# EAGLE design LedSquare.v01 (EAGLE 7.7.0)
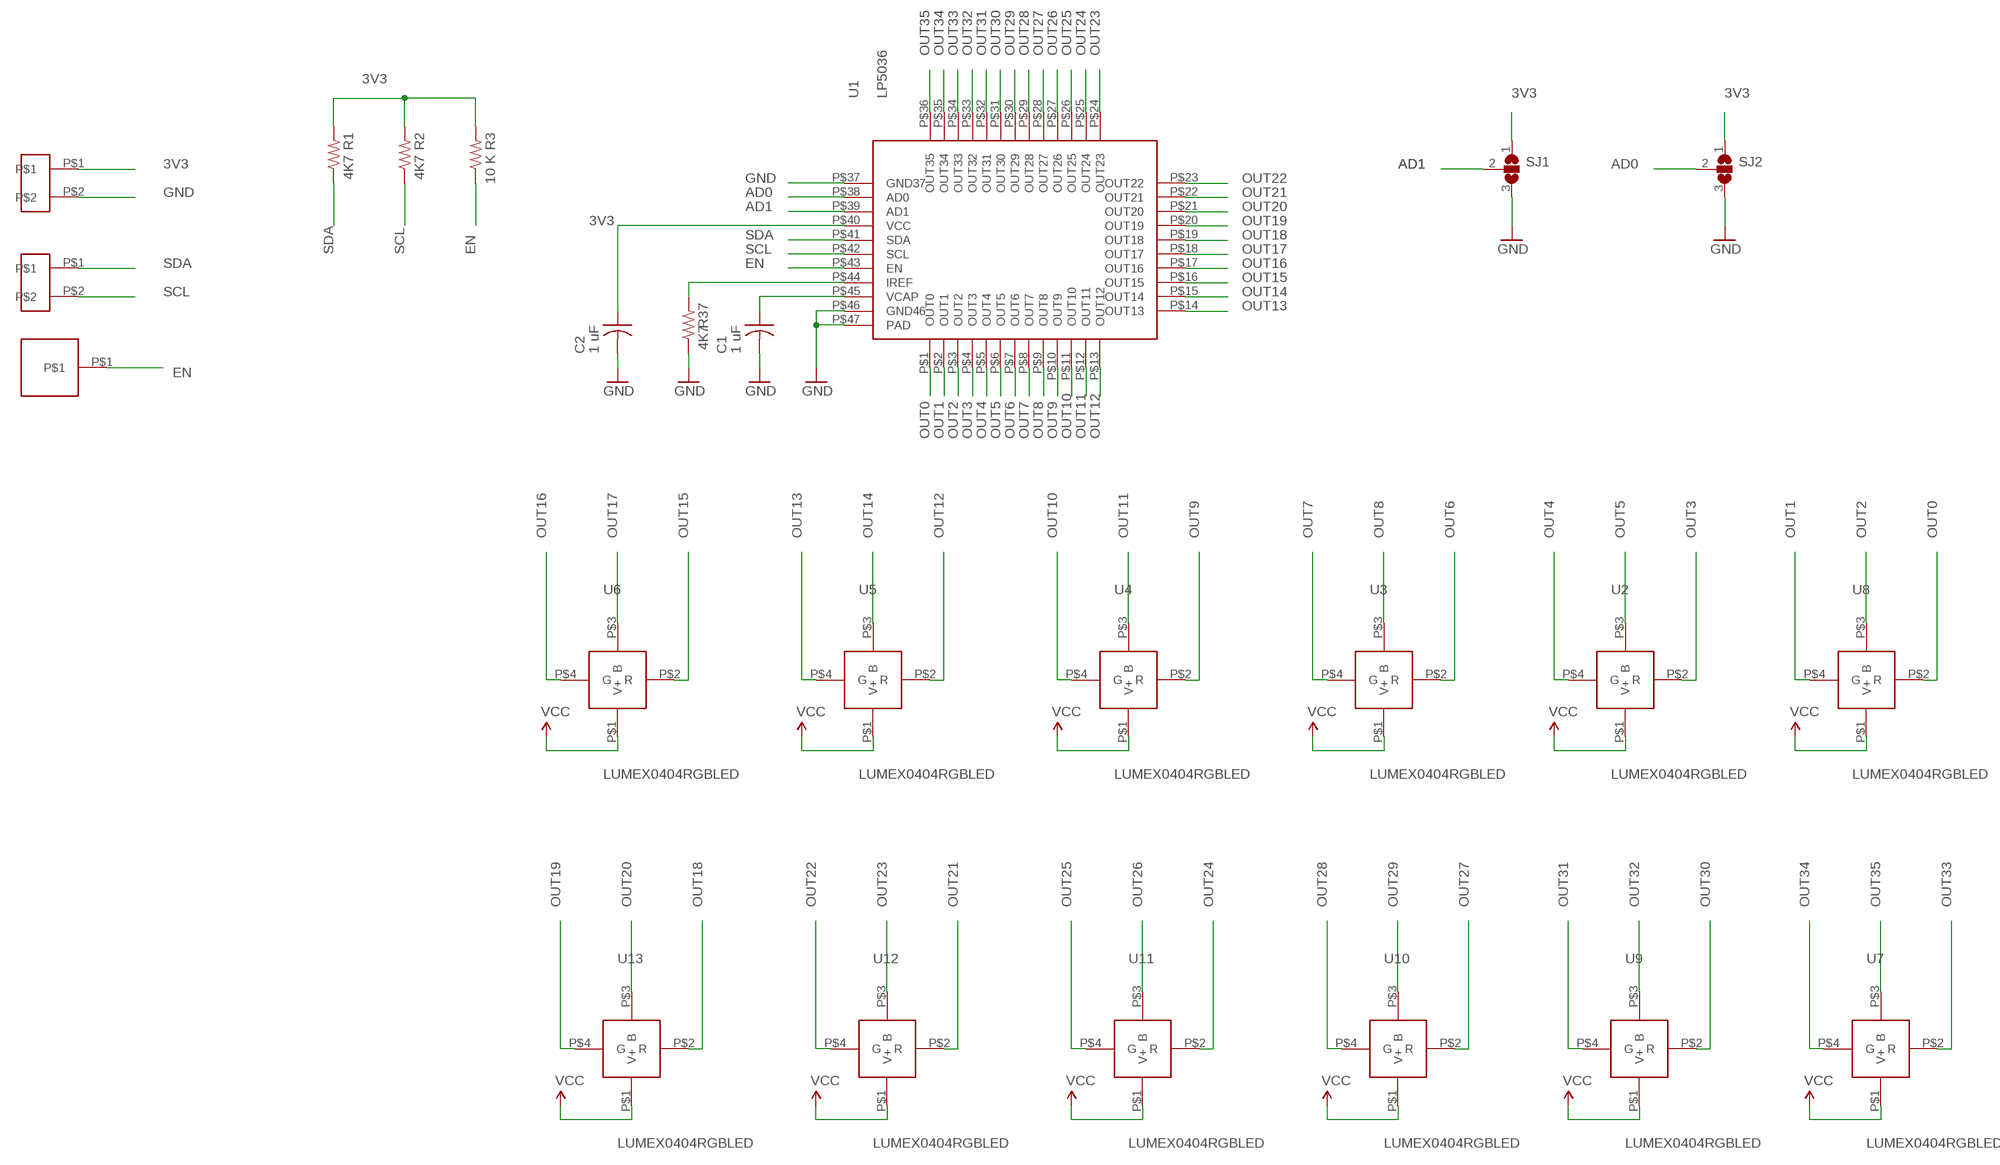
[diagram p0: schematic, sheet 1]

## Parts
C1  1 uF  C-US  [C0402_B]
C2  1 uF  C-US  [C0402_B]
R1  4K7  R-US_  [R0402_B]
R2  4K7  R-US_  [R0402_B]
R3  10 K  R-US_  [R0402_B]
R37  4K7  R-US_  [R0402_B]
SJ1  SJ2W  [SJ_2]
SJ2  SJ2W  [SJ_2]
U1  LP5036  [LP5036]
U2  LUMEX0404RGBLED  [LX0404]
U3  LUMEX0404RGBLED  [LX0404]
U4  LUMEX0404RGBLED  [LX0404]
U5  LUMEX0404RGBLED  [LX0404]
U6  LUMEX0404RGBLED  [LX0404]
U7  LUMEX0404RGBLED  [LX0404]
U8  LUMEX0404RGBLED  [LX0404]
U9  LUMEX0404RGBLED  [LX0404]
U10  LUMEX0404RGBLED  [LX0404]
U11  LUMEX0404RGBLED  [LX0404]
U12  LUMEX0404RGBLED  [LX0404]
U13  LUMEX0404RGBLED  [LX0404]
U$9  HN01  [HN01]
U$17  HN02  [HN02]
U$39  HN02  [HN02]

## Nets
3V3: C2.1 R1.2 R2.2 R3.2 SJ1.1 SJ2.1 U1.P$40(VCC) U2.P$1(V+) U3.P$1(V+) U4.P$1(V+) U5.P$1(V+) U6.P$1(V+) U7.P$1(V+) U8.P$1(V+) U9.P$1(V+) U10.P$1(V+) U11.P$1(V+) U12.P$1(V+) U13.P$1(V+) U$39.P$1 ; supply symbol labelled VCC
AD0: SJ2.2 U1.P$38(AD0)
AD1: SJ1.2 U1.P$39(AD1)
EN: R3.1 U1.P$43(EN) U$9.P$1
GND: C1.2 C2.2 R37.1 SJ1.3 SJ2.3 U1.P$37(GND37) U1.P$46(GND46) U1.P$47(PAD) U$39.P$2
N$80: R37.2 U1.P$44(IREF)
N$81: C1.1 U1.P$45(VCAP)
OUT0: U1.P$1(OUT0) U8.P$2(R)
OUT1: U1.P$2(OUT1) U8.P$4(G)
OUT2: U1.P$3(OUT2) U8.P$3(B)
OUT3: U1.P$4(OUT3) U2.P$2(R)
OUT4: U1.P$5(OUT4) U2.P$4(G)
OUT5: U1.P$6(OUT5) U2.P$3(B)
OUT6: U1.P$7(OUT6) U3.P$2(R)
OUT7: U1.P$8(OUT7) U3.P$4(G)
OUT8: U1.P$9(OUT8) U3.P$3(B)
OUT9: U1.P$10(OUT9) U4.P$2(R)
OUT10: U1.P$11(OUT10) U4.P$4(G)
OUT11: U1.P$12(OUT11) U4.P$3(B)
OUT12: U1.P$13(OUT12) U5.P$2(R)
OUT13: U1.P$14(OUT13) U5.P$4(G)
OUT14: U1.P$15(OUT14) U5.P$3(B)
OUT15: U1.P$16(OUT15) U6.P$2(R)
OUT16: U1.P$17(OUT16) U6.P$4(G)
OUT17: U1.P$18(OUT17) U6.P$3(B)
OUT18: U1.P$19(OUT18) U13.P$2(R)
OUT19: U1.P$20(OUT19) U13.P$4(G)
OUT20: U1.P$21(OUT20) U13.P$3(B)
OUT21: U1.P$22(OUT21) U12.P$2(R)
OUT22: U1.P$23(OUT22) U12.P$4(G)
OUT23: U1.P$24(OUT23) U12.P$3(B)
OUT24: U1.P$25(OUT24) U11.P$2(R)
OUT25: U1.P$26(OUT25) U11.P$4(G)
OUT26: U1.P$27(OUT26) U11.P$3(B)
OUT27: U1.P$28(OUT27) U10.P$2(R)
OUT28: U1.P$29(OUT28) U10.P$4(G)
OUT29: U1.P$30(OUT29) U10.P$3(B)
OUT30: U1.P$31(OUT30) U9.P$2(R)
OUT31: U1.P$32(OUT31) U9.P$4(G)
OUT32: U1.P$33(OUT32) U9.P$3(B)
OUT33: U1.P$34(OUT33) U7.P$2(R)
OUT34: U1.P$35(OUT34) U7.P$4(G)
OUT35: U1.P$36(OUT35) U7.P$3(B)
SCL: R2.1 U1.P$42(SCL) U$17.P$2
SDA: R1.1 U1.P$41(SDA) U$17.P$1

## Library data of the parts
C1 C2 = Spark:C-US: Capacitor
R1-R3 R37 = Spark:R-US_: 0402 Resistor
SJ1 SJ2 = jumper:SJ2W: SMD solder JUMPER
U1 = Kris:LP5036: LP5036RJVR 12 x 3 rgb led driver http://www.ti.com/lit/ds/symlink/lp5036.pdf
U2-U13 = Kris:LUMEX0404RGBLED: Lumex 0404 rgb leds
U$9 = PWSONN6:HN01
U$17 U$39 = Kris:HN02: 0.1 inch header

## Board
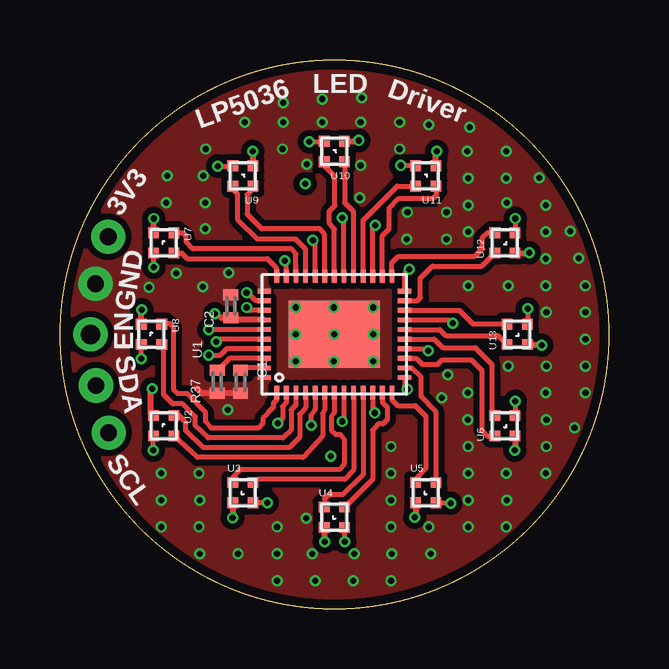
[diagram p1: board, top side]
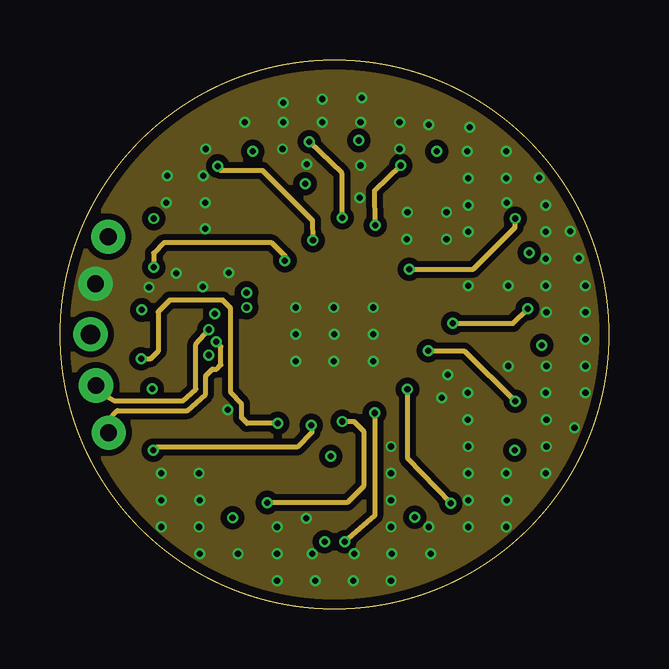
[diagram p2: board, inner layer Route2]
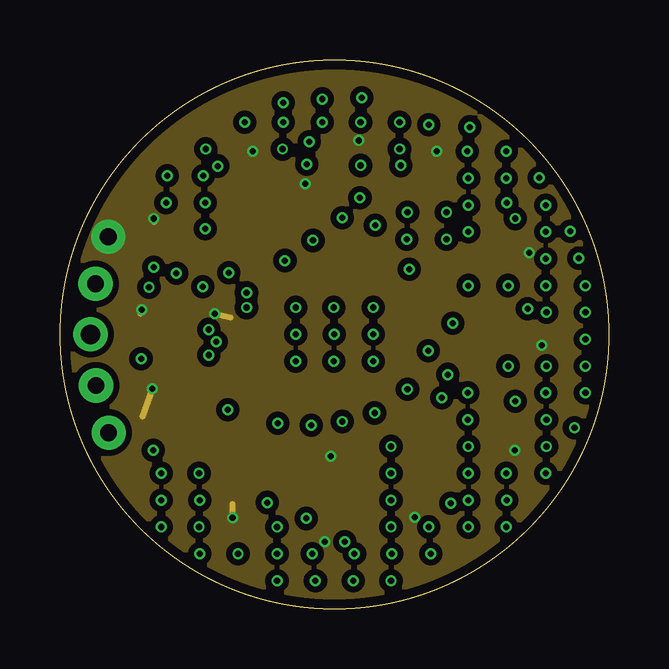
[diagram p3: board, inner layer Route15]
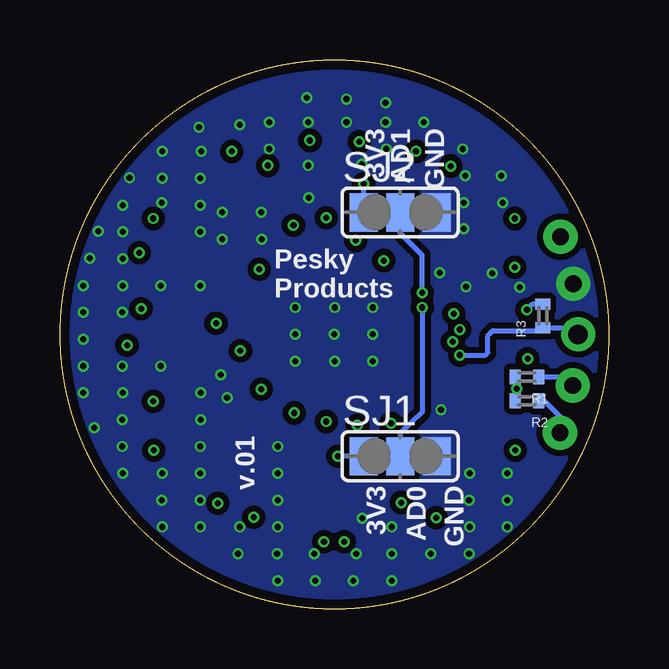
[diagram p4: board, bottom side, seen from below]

Size 22.86 x 22.86 mm. Coordinates in mm from the lower left corner, seen from the top.
Outline: circle at 11.43,11.43 radius 11.43
Copper layers (1*2*15*16): Top 0.035559375mm / dielectric 0.17018125mm / Route2 0.01778125mm / dielectric 47mil / Route15 0.01778125mm / dielectric 0.17018125mm / Bottom 0.035559375mm
Design rules "OSHPark-4layer *": minimum track width 5mil, minimum drill 10mil, track to track 5mil, track to pad 5mil, pad to pad 5mil, via to via 5mil, smd to smd 5mil, copper to edge 15mil, drill to drill 6mil, minimum pad ring 4mil, minimum via ring 4mil, stop-mask expansion 4mil, vias tented up to drill 20mil, thermal gap 10mil

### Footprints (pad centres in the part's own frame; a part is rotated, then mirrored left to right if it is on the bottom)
C0402_B = smd 0.457 x 0.61: 1 -0.483,0; 2 0.483,0
R0402_B = smd 0.457 x 0.61: 1 -0.483,0; 2 0.483,0
SJ_2 = smd 1.168 x 1.6: 1 -1.524,0; 2 0,0; 3 1.524,0
LP5036 = smd 0.55 x 0.2: P$1 -2.425,2.4; P$2 -2.425,2; P$3 -2.425,1.6; P$4 -2.425,1.2; P$5 -2.425,0.8; P$6 -2.425,0.4; P$7 -2.425,0; P$8 -2.425,-0.4; P$9 -2.425,-0.8; P$10 -2.425,-1.2; P$11 -2.425,-1.6; P$12 -2.425,-2; P$13 -2.425,-2.4; P$24 2.425,-2.4; P$25 2.425,-2; P$26 2.425,-1.6; P$27 2.425,-1.2; P$28 2.425,-0.8; P$29 2.425,-0.4; P$30 2.425,0; P$31 2.425,0.4; P$32 2.425,0.8; P$33 2.425,1.2; P$34 2.425,1.6; P$35 2.425,2; P$36 2.425,2.4 | smd 0.2 x 0.55: P$14 -1.8,-2.925; P$15 -1.4,-2.925; P$16 -1,-2.925; P$17 -0.6,-2.925; P$18 -0.2,-2.925; P$19 0.2,-2.925; P$20 0.6,-2.925; P$21 1,-2.925; P$22 1.4,-2.925; P$23 1.8,-2.925; P$37 1.8,2.925; P$38 1.4,2.925; P$39 1,2.925; P$40 0.6,2.925; P$41 0.2,2.925; P$42 -0.2,2.925; P$43 -0.6,2.925; P$44 -1,2.925; P$45 -1.4,2.925; P$46 -1.8,2.925 | smd 2.8 x 3.8: P$47 0,0
LX0404 = smd 0.45 x 0.45: P$1 -0.425,-0.425; P$2 -0.425,0.425; P$3 0.425,0.425; P$4 0.425,-0.425
HN01 = drill 0.813 pad 1.422: P$1 0,0
HN02 = drill 0.7 pad 1.422: P$1 0,0; P$2 -2.032,0

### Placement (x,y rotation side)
C1  7.52,9.45 270 top
C2  7.11,12.6 90 top
R1  3.4,9.65 180 bottom
R2  3.4,8.66 180 bottom
R3  2.74,12.19 90 bottom
R37  6.55,9.45 90 top
SJ1  8.69,6.35 0 bottom
SJ2  8.69,16.51 0 bottom
U1  11.43,11.43 90 top
U2  4.32,7.62 270 top
U3  7.62,4.83 0 top
U4  11.43,3.81 0 top
U5  15.24,4.83 0 top
U6  18.54,7.62 90 top
U7  4.32,15.24 270 top
U8  3.81,11.43 270 top
U9  7.62,18.03 180 top
U10  11.43,19.05 180 top
U11  15.24,18.03 180 top
U12  18.54,15.24 90 top
U13  19.05,11.43 90 top
U$9  1.27,11.43 0 top
U$17  1.5,9.3 105 top
U$39  2.01,15.49 75 top

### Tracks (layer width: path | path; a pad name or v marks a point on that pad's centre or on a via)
3V3  (via drill 0.25)
  Top 0.254: U1.P$40 7.23,12.03 C2.1 6.73,12.12 v6.45,12.29 | U9.P$1 8.04,19.03 v8.03,19.05 | U10.P$1 12.53,19.48 v12.45,19.51 | U11.P$1 15.66,18.98 v15.7,19.05 | U12.P$1 19.49,14.82 v19.56,14.83 | U13.P$1 20.03,11.01 v20.07,10.97 | U6.P$1 18.96,6.62 v18.95,6.6 | U5.P$1 14.82,3.88 v14.78,3.81 | U4.P$1 11.01,2.86 v11.02,2.79 | U8.P$1 3.39,12.43 v3.4,12.45 | U7.P$1 3.9,16.14 v3.91,16.26 | U3.P$1 7.2,3.74 v7.19,3.79 | U2.P$1 3.87,8.04 3.79,8.13 3.79,9.11 v3.84,9.16
  Route15 0.203: v11.28,6.35 11.38,6.4
  Route15 0.254: v6.45,12.29 7.11,12.14 | v8.03,19.05 8.03,19.1 8.08,19.05 | v12.45,19.51 12.39,19.46 12.34,19.51 | v15.7,19.05 15.65,18.95 | v19.56,14.83 19.51,14.83 | v20.07,10.97 19.96,10.97 20.02,11.02 | v18.95,6.6 18.95,6.71 | v14.78,3.81 14.83,3.86 14.78,3.91 | v11.02,2.79 10.97,2.79 | v3.84,9.16 3.43,8 | v3.4,12.45 3.45,12.39 3.35,12.29 | v3.91,16.26 3.96,16.15 3.91,16.1 | v7.19,3.79 7.19,4.37
  Bottom 0.203: SJ2.1 v10.21,17.7 | SJ1.1 v11.28,6.35 11.38,6.35 | R3.2 3.18,12.68 v3.4,12.45 | R2.2 3.86,9.13 v3.84,9.16
  Bottom 0.254: R1.2 R2.2
  pour Route15 (isolate 0.254, no thermals): -1.27,24.13 24.13,24.13 24.13,-1.27 -1.27,-1.27
AD0  (via drill 0.25)
  Top 0.203: U1.P$38 8.15,12.83 7.82,13.16 v7.77,13.16
  Bottom 0.203: v7.77,13.16 7.77,14.73 8.69,15.65 SJ2.2
AD1  (via drill 0.25)
  Top 0.203: U1.P$39 7.94,12.43 v7.77,12.55
  Bottom 0.127: SJ1.2 7.21,6.35
  Bottom 0.203: v7.77,12.55 7.77,8.18 8.69,7.32 SJ1.2
EN  (via drill 0.25)
  Top 0.203: U1.P$43 6.94,10.83 6.68,10.57 v6.2,10.57
  Bottom 0.203: v6.2,10.57 5.13,10.57 5.03,10.67 5.03,11.38 4.83,11.58 2.95,11.58 R3.1 1.55,11.71 U$9.P$1
GND  (via drill 0.25)
  Top 0.254: C1.2 5.92,8.97 5.72,9.17
  other vias: 11.43,11.43 6.99,8.28 9.83,12.55 11.4,12.55 13.06,12.55 13.06,10.31 13.06,11.43 11.4,10.31 9.83,10.31 9.83,11.43 5.82,4.52 4.22,5.64 5.79,5.64 5.79,3.4 4.22,3.4 4.22,4.52 7.42,2.29 9.04,3.4 9.04,1.17 9.04,2.29 5.82,2.29 10.64,1.17 10.52,2.29 12.27,2.29 13.82,2.29 13.79,3.4 15.44,2.29 13.79,1.17 12.22,1.17 13.79,5.64 17.02,5.64 17.02,3.4 17.02,4.52 15.37,3.4 13.79,4.52 13.79,6.76 17.02,6.76 18.62,4.52 18.59,5.64 20.24,5.64 18.59,3.4 16.99,8.99 20.27,6.76 20.27,7.87 16.99,7.87 20.27,10.11 21.89,11.23 21.89,8.99 21.89,10.11 20.24,8.99 18.67,10.11 20.27,12.34 18.67,13.46 20.24,13.46 21.89,13.46 21.89,12.34 16.15,9.75 15.9,8.79 17.02,15.7 20.24,15.7 20.24,14.58 17.02,13.46 18.62,16.92 17.02,17.93 18.59,17.93 20.24,16.81 17.02,16.81 16.97,19.05 15.37,20.17 17.07,20.07 18.59,19.05 19.96,17.96 21.62,14.61 21.26,15.72 6.07,19.15 7.04,14 7.7,20.27 5.97,18.03 4.47,18.03 4.42,16.92 6.05,15.82 6.05,16.92 9.3,20.27 9.3,21.08 10.92,21.23 10.92,20.27 9.27,19.15 12.52,20.27 12.57,21.29 14.15,19.15 14.15,20.27 14.48,16.51 16.1,15.39 16.1,16.51 14.45,15.39 12.52,18.47 12.5,17.12 5.94,13.41 4.85,13.97 3.71,13.39 10.29,18.52 21.44,7.54 10.26,3.76
  pour Bottom (isolate 0.254, no thermals): -1.27,24.13 24.13,24.13 24.13,-1.27 -1.27,-1.27
  pour Top (isolate 0.254, no thermals): -1.27,24.13 24.13,24.13 24.13,-1.27 -1.27,-1.27
  pour Route2 (isolate 0.254, no thermals): -1.27,24.13 24.13,24.13 24.13,-1.27 -1.27,-1.27
N$2
  Bottom 0.127: 8.69,16.51 7.21,16.51
N$80
  Top 0.203: U1.P$44 7.08,10.43 6.55,9.91 6.43,9.91 R37.2
N$81
  Top 0.203: U1.P$45 7.67,10.03 C1.1
OUT0
  Top 0.203: U1.P$1 9.03,8.7 8.89,8.56 8.89,8.38 8.66,8.15 8.59,8.05 8.46,7.93 8.46,7.72 8.26,7.52 6.3,7.52 6.07,7.8 6.07,8.15 5.28,8.97 4.9,8.97 4.72,9.14 4.72,11.71 4.57,11.89 4.27,11.89 U8.P$2
OUT1  (via drill 0.25)
  Top 0.203: U1.P$2 9.43,8.59 9.27,8.43 9.27,7.93 v9.07,7.72 | v3.38,10.41 3.38,10.67 U8.P$4
  Route2 0.203: v9.07,7.72 7.8,7.72 7.57,7.95 7.57,8.53 7.11,9.02 7.11,12.52 6.78,12.85 4.57,12.85 4.09,12.37 4.09,10.72 3.79,10.41 v3.38,10.41
OUT2
  Top 0.203: U1.P$3 9.83,8.48 9.63,8.28 9.63,7.44 9.3,7.11 6.17,7.11 5.64,7.62 5.64,8 5.11,8.53 4.7,8.53 4.32,8.92 4.32,10.73 U8.P$3
OUT3
  Top 0.203: U1.P$4 10.23,8.38 9.98,8.1 9.98,7.14 9.55,6.71 5.97,6.71 5.23,7.42 5.23,7.77 4.98,8.05 4.78,8.05 U2.P$2
OUT4  (via drill 0.25)
  Top 0.203: U1.P$5 10.63,8.29 10.46,8.08 v10.46,7.64 | v3.89,6.6 3.89,7.18 U2.P$4
  Route2 0.203: v10.46,7.64 10.49,7.34 9.88,6.73 4.04,6.73 v3.89,6.6
OUT5
  Top 0.203: U1.P$6 11.03,8.29 10.95,8.13 10.95,7.21 10.13,6.3 5.72,6.3 U2.P$3
OUT6
  Top 0.203: U1.P$7 11.43,8.18 11.3,8 11.3,7.44 11.48,7.26 11.68,7.26 11.84,7.06 11.84,6.02 11.63,5.79 7.49,5.79 7.21,5.49 7.24,5.3 U3.P$2 7.21,5.27
OUT7  (via drill 0.25)
  Top 0.203: U1.P$8 11.83,7.92 v11.76,7.8 | v8.64,4.42 U3.P$4
  Route2 0.203: 8.71,4.47 v8.64,4.42 11.96,4.42 12.65,5.11 12.65,7.39 12.24,7.8 v11.76,7.8
OUT8
  Top 0.203: U3.P$3 8.22,5.39 11.86,5.39 12.23,5.78 U1.P$9
OUT9
  Top 0.203: U4.P$2 11.02,4.25 11.02,4.57 11.2,4.75 11.79,4.75 12.63,5.57 U1.P$10
OUT10  (via drill 0.25)
  Top 0.203: U1.P$11 13.03,8.2 v13.11,8.15 | v11.86,2.79 11.86,3.38 U4.P$4
  Route2 0.203: v13.11,8.15 13.11,3.86 v11.86,2.79
OUT11
  Top 0.203: 11.87,4.22 U4.P$3 13.03,5.39 13.03,7.44 13.26,7.7 13.46,7.7 13.64,7.87 13.64,8.38 13.43,8.59 U1.P$12
OUT12
  Top 0.203: U1.P$13 13.83,8.7 14.07,8.46 14.81,8.46 15.24,8.03 15.24,5.84 14.81,5.39 14.81,5.26 U5.P$2
OUT13  (via drill 0.25)
  Top 0.203: U1.P$14 14.36,9.27 v14.48,9.14 | v16.28,4.39 15.68,4.39 U5.P$4
  Route2 0.203: v14.48,9.14 14.48,6.27 v16.28,4.39
OUT14
  Top 0.203: U1.P$15 14.66,10.03 15.04,9.68 15.04,8.84 15.65,8.2 15.65,5.27 U5.P$3
OUT15
  Top 0.203: U1.P$16 14.84,10.43 15.09,10.19 15.75,10.19 15.93,10.36 17.14,10.36 17.58,9.93 17.58,7.44 17.8,7.19 U6.P$2
OUT16  (via drill 0.25)
  Top 0.203: U1.P$17 15.26,10.83 v15.34,10.74 | v18.97,8.64 18.97,8.06 U6.P$4
  Route2 0.203: v15.34,10.74 16.84,10.74 v18.97,8.64
OUT17
  Top 0.203: U1.P$18 15.59,11.23 15.95,10.87 17.3,10.87 17.98,10.19 17.98,8.1 U6.P$3
OUT18
  Top 0.203: U1.P$19 15.83,11.63 16.08,11.38 18.25,11.38 U13.P$2
OUT19  (via drill 0.25)
  Top 0.203: U1.P$20 16.21,12.03 v16.36,11.89 | v19.48,12.5 19.48,11.86 U13.P$4
  Route2 0.203: v16.36,11.89 18.87,11.89 v19.48,12.5
OUT20
  Top 0.203: U1.P$21 16.64,12.43 17.21,11.86 U13.P$3
OUT21
  Top 0.203: U1.P$22 14.89,12.83 15.01,12.95 15.01,13.77 15.52,14.28 17.57,14.28 U12.P$2
OUT22  (via drill 0.25)
  Top 0.203: U1.P$23 14.36,13.95 v14.55,14.15 | v18.97,16.26 18.97,15.68 U12.P$4
  Route2 0.203: v14.55,14.15 17.22,14.15 18.95,15.88 18.95,16.23 v18.97,16.26
OUT23
  Top 0.203: U1.P$24 13.83,14.41 14.1,14.68 17.27,14.68 17.6,14.99 17.6,15.47 17.8,15.67 U12.P$3
OUT24
  Top 0.203: U11.P$2 15.7,17.57 15.7,17.25 15.55,17.09 14.12,17.09 13.72,16.69 13.72,15.82 13.43,15.54 U1.P$25
OUT25  (via drill 0.25)
  Top 0.203: U1.P$26 13.03,15.85 v13.13,15.98 | v14.2,18.47 14.8,18.47 U11.P$4
  Route2 0.203: v13.13,15.98 13.11,17.42 v14.2,18.47
OUT26
  Top 0.203: U1.P$27 12.63,16.19 14.05,17.6 U11.P$3
OUT27
  Top 0.203: U1.P$28 12.23,16.54 11.86,16.91 U10.P$2
OUT28  (via drill 0.25)
  Top 0.203: U1.P$29 11.83,16.11 v11.76,16.28 | v10.39,19.46 10.99,19.46 U10.P$4
  Route2 0.203: v11.76,16.28 11.76,18.14 v10.39,19.46
OUT29
  Top 0.203: U1.P$30 11.43,15.82 11.23,16.05 11.23,16.56 11.46,16.79 11.46,18.01 11.02,18.44 11.02,18.61 U10.P$3
OUT30
  Top 0.203: U1.P$31 11.03,15.59 10.85,15.82 8.41,15.82 7.8,16.43 7.8,17.25 8.03,17.5 8.03,17.59 U9.P$2
OUT31  (via drill 0.25)
  Top 0.203: U1.P$32 10.63,15.23 v10.54,15.34 | v6.58,18.44 U9.P$4
  Route2 0.203: v6.58,18.44 6.68,18.26 8.43,18.26 10.52,16.18 v10.54,15.34
OUT32
  Top 0.203: U1.P$33 10.23,14.97 9.83,15.39 8.23,15.39 7.39,16.23 7.39,17.27 7.19,17.48 U9.P$3
OUT33
  Top 0.203: U1.P$34 9.83,14.15 9.83,14.28 9.83,14.78 9.65,14.99 5.54,14.99 5.26,15.29 5.26,15.52 5.13,15.65 4.77,15.65 U7.P$2
OUT34  (via drill 0.25)
  Top 0.203: U1.P$35 9.43,14.39 v9.37,14.5 | v3.91,14.22 3.91,14.8 U7.P$4
  Route2 0.203: v9.37,14.5 9.37,14.71 8.81,15.24 4.32,15.24 U7.P$4 3.9,14.09 v3.91,14.22
OUT35
  Top 0.203: U1.P$36 9.03,14.19 8.64,14.58 5.31,14.58 5.07,14.82 U7.P$3
SCL  (via drill 0.25)
  Top 0.203: U1.P$42 8.33,11.23 6.71,11.23 v6.5,11.12
  Route2 0.203: U$17.P$2 2.03,7.87 2.39,8.26 5.31,8.26 6.07,8.94 6.07,9.7 6.35,9.98 6.53,9.98 6.71,10.16 6.71,10.92 v6.5,11.12
  Bottom 0.203: R2.1 2.69,8.66 2.03,8.03 2.03,7.34 U$17.P$2
SDA  (via drill 0.25)
  Top 0.203: U1.P$41 v6.2,11.63
  Route2 0.203: v6.19,11.63 v6.2,11.63 5.66,11.02 5.66,9.14 5.11,8.66 2.26,8.66 1.65,8.99 U$17.P$1
  Bottom 0.203: R1.1 1.98,9.65 U$17.P$1

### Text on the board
tPlace: LED | Driver | LP5036 | 3V3 | GND | EN | SDA | SCL
bPlace: GND | AD1 | 3V3 | Pesky / Products | v.01 | GND | AD0 | 3V3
